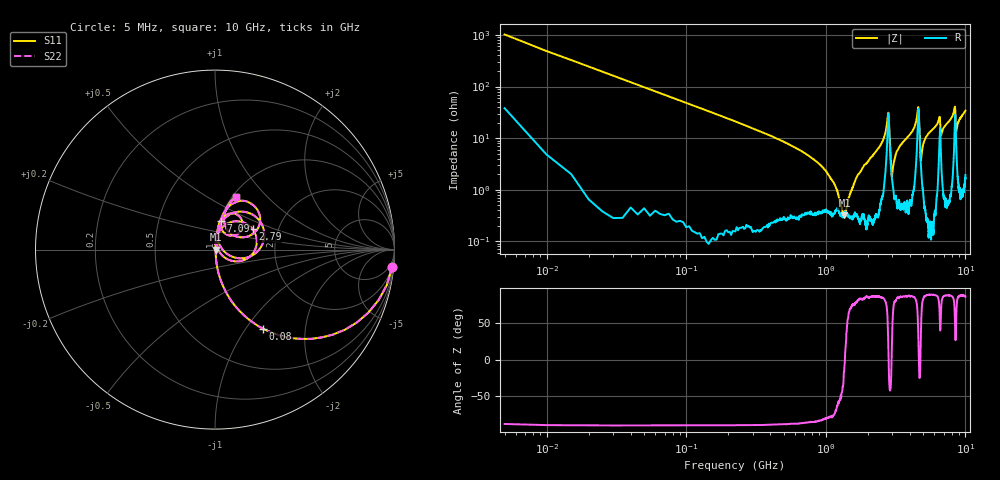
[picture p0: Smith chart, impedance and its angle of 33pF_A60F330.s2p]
! Amotech Co.,Ltd.
! http://www.amotech.co.kr/
! Part Number: A60F330
! These Parameters are Measured in Series Mode Connection
! Operation Temp=25[degC], DC Bias Voltage=0[V]
! Freq. Start=5[MHz] Stop=10[GHz], 2000[Steps]
! Date: Monday, July 20, 2020, 03:40:01
# GHZ S RI R 50.000000
!Freq.(Hz) S11(Real) S11(Imag) S21(Real) S21(Imag) S12(Real) S12(Imag) S22(Real) S22(Imag)
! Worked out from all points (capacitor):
!   2000 points, 5 MHz to 10 GHz, reference 50 ohm
!   read as one part in series: C = 32.9 pF near 55 MHz
!   lowest |Z| = 321 mohm at 1.36 GHz (marker M1)
!   series resonance near 1.371 GHz, so ESL is about 410 pH
!   S11 on the Smith chart (normalised r, x): 5 MHz: 2, -20; 80 MHz: 1.01, -1.21; 2.79 GHz: 1.48, +0.36; 7.09 GHz: 1.01, +0.34; 10 GHz: 1.04, +0.68
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0.005  0.9869 -0.0966  0.0131 0.0966  0.0131 0.0966  0.9869 -0.0966
0.08  0.268 -0.4407  0.732 0.4407  0.732 0.4407  0.268 -0.4407
0.265  0.0319 -0.1706  0.9681 0.1706  0.9681 0.1706  0.0319 -0.1706
0.99  0.00462 -0.0234  0.9954 0.0234  0.9954 0.0234  0.00462 -0.0234
1.36  0.00316 -0.000459  0.9968 0.000459  0.9968 0.000459  0.00316 -0.000459
1.675  0.00353 0.0179  0.9965 -0.0179  0.9965 -0.0179  0.00353 0.0179
2.55  0.015 0.0851  0.985 -0.0851  0.985 -0.0851  0.015 0.0851
2.79  0.209 0.1152  0.791 -0.1152  0.791 -0.1152  0.209 0.1152
2.835  0.1646 -0.0575  0.8354 0.0575  0.8354 0.0575  0.1646 -0.0575
2.975  0.0168 0.00614  0.9832 -0.00614  0.9832 -0.00614  0.0168 0.00614
3.34  0.0105 0.0637  0.9895 -0.0637  0.9895 -0.0637  0.0105 0.0637
4.33  0.0395 0.1584  0.9605 -0.1584  0.9605 -0.1584  0.0395 0.1584
4.575  0.2364 0.1743  0.7636 -0.1743  0.7636 -0.1743  0.2364 0.1743
4.64  0.229 -0.0176  0.771 0.0176  0.771 0.0176  0.229 -0.0176
4.79  0.0316 0.0153  0.9684 -0.0153  0.9684 -0.0153  0.0316 0.0153
5.005  0.0136 0.0769  0.9864 -0.0769  0.9864 -0.0769  0.0136 0.0769
6.5  0.1085 0.2003  0.8915 -0.2003  0.8915 -0.2003  0.1085 0.2003
6.67  0.0622 0.0857  0.9378 -0.0857  0.9378 -0.0857  0.0622 0.0857
7.09  0.034 0.1621  0.966 -0.1621  0.966 -0.1621  0.034 0.1621
8.335  0.1749 0.2689  0.8251 -0.2689  0.8251 -0.2689  0.1749 0.2689
8.595  0.0783 0.0962  0.9217 -0.0962  0.9217 -0.0962  0.0783 0.0962
10  0.1166 0.2938  0.8834 -0.2938  0.8834 -0.2938  0.1166 0.2938
